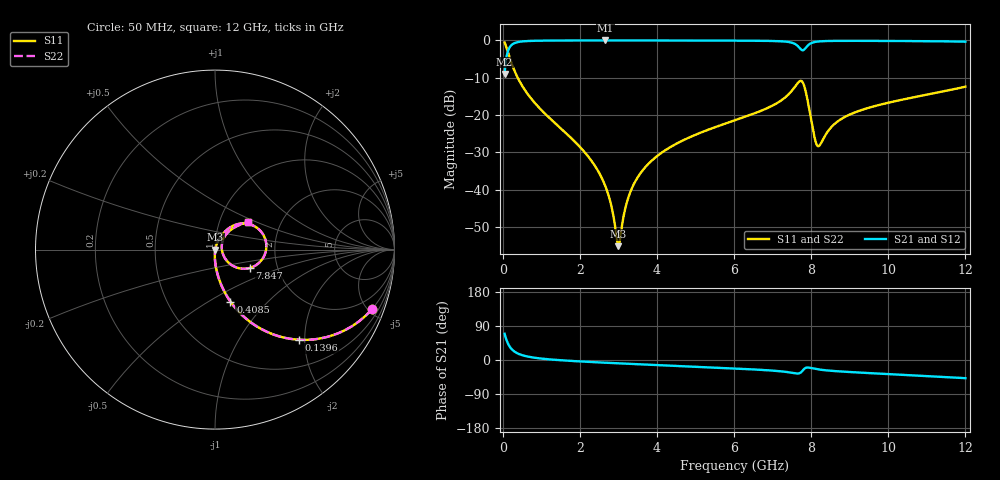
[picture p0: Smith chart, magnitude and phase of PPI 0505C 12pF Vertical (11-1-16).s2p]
# GHz S MA R 50
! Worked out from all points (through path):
!   1601 points, 50 MHz to 12 GHz, reference 50 ohm
!   highest |S21| = -0.02 dB at 2.664 GHz (marker M1); lowest = -9.0 dB at 50 MHz (marker M2)
!   group delay of S21, straight-line fit = 13.4 ps
!   lowest |S11| = -55.2 dB at 3 GHz (marker M3), VSWR 1.00, Z = 50.2 - j0.035 ohm
!   |S11| at or under -10 dB: 389.7 MHz to end of sweep
!   |S22| runs from -55.2 to -0.6 dB; largest |S21 - S12| = 0
!   S11 on the Smith chart (normalised r, x): 50 MHz: 0.99, -5.25; 139.6 MHz: 0.99, -1.88; 408.5 MHz: 0.99, -0.63; 7.847 GHz: 1.44, -0.31; 12 GHz: 1.37, +0.45
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0.05  0.9352 -20.9  0.354 69.1  0.354 69.1  0.9352 -20.9
0.139625  0.6864 -47.0  0.7269 42.9  0.7269 42.9  0.6864 -47.0
0.2516563  0.4621 -63.2  0.8863 26.8  0.8863 26.8  0.4621 -63.2
0.4085  0.3026 -73.5  0.9524 16.4  0.9524 16.4  0.3026 -73.5
0.94625  0.1252 -85.1  0.9911 4.4  0.9911 4.4  0.1252 -85.1
2.044156  0.03542 -91.6  0.9978 -4.0  0.9978 -4.0  0.03542 -91.6
2.664062  0.01108 -88.7  0.9981 -7.2  0.9981 -7.2  0.01108 -88.7
3.000156  0.001747 -11.5  0.9981 -8.8  0.9981 -8.8  0.001747 -11.5
3.209281  0.006443 63.9  0.998 -9.8  0.998 -9.8  0.006443 63.9
3.373594  0.01107 69.8  0.9979 -10.5  0.9979 -10.5  0.01107 69.8
4.038312  0.02902 72.4  0.9972 -13.5  0.9972 -13.5  0.02902 72.4
6.025  0.08509 65.3  0.9926 -22.4  0.9926 -22.4  0.08509 65.3
7.04075  0.1373 57.7  0.9806 -28.3  0.9806 -28.3  0.1373 57.7
7.548625  0.2276 39.5  0.9125 -34.5  0.9125 -34.5  0.2276 39.5
7.727875  0.2873 7.6  0.7644 -33.2  0.7644 -33.2  0.2873 7.6
7.847375  0.2184 -28.0  0.7822 -21.3  0.7822 -21.3  0.2184 -28.0
8.019156  0.07636 -41.6  0.9273 -21.7  0.9273 -21.7  0.07636 -41.6
8.11625  0.04373 -19.5  0.9559 -23.7  0.9559 -23.7  0.04373 -19.5
8.198406  0.0384 10.7  0.968 -25.0  0.968 -25.0  0.0384 10.7
8.795906  0.08943 53.6  0.9862 -30.5  0.9862 -30.5  0.08943 53.6
10.01331  0.1466 50.7  0.9831 -37.2  0.9831 -37.2  0.1466 50.7
12  0.2399 39.8  0.9612 -48.1  0.9612 -48.1  0.2399 39.8
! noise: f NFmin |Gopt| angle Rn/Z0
0.05  0.0004026  0.8728  1.599  0.0006822
1.372  0.004104  0.682  4.36  0.002496
2.701  0.006798  0.6335  7.985  0.003473
4.031  0.009324  0.6085  11.59  0.004369
5.36  0.01223  0.6056  15.16  0.005639
6.682  0.01926  0.6758  18.91  0.01117
8.012  0.07931  0.8939  23.19  0.1564
9.341  0.02463  0.6545  26.26  0.01291
10.67  0.02453  0.6161  29.34  0.01117
12  0.03297  0.6707  33.01  0.01777
